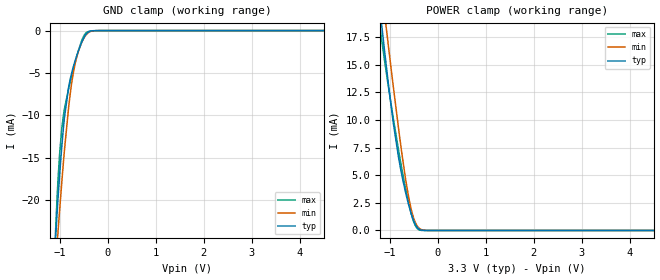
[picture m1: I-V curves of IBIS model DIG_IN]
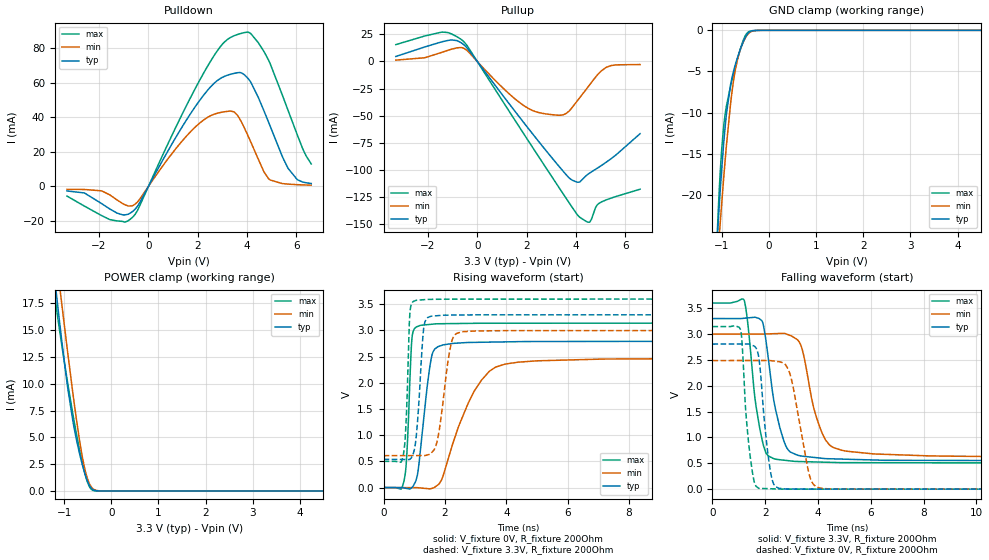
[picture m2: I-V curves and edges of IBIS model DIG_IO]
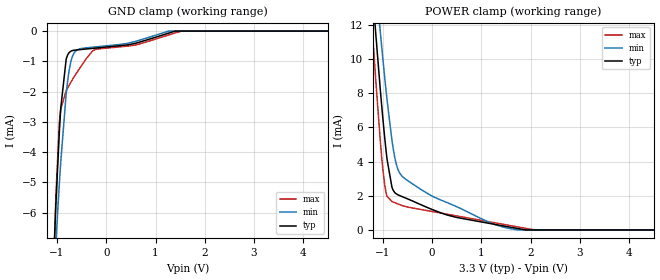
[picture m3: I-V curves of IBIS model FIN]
|Texas Instruments Incorporated
| 13.5 GHz Low Phase Noise Fractional N PLL with Ramp/Chirp Generation
| Part#   Digital Voltage Range   Package-type   #pins
| LMX2492Q   3.0V - 3.6V   PQFP   24
[IBIS Ver]   4.1
[File name]   lmx2492q.ibs
[File Rev]   1.0
[Date]   03/11/2014
[Source]
| Texas Instruments Incorporated.
| 12500 TI Blvd
| Dallas, TX -75243
[Notes]   Revision History:
| Rev 1.0: 03/11/2014
| - Initial version of the model
| - Model generated from simulations in TISPICE
| - C_comp although listed in numerical order of value are
|   obtained from varying PVT conditions. For PVT conditions for
|   each specific value refer the buffer description under
|   respective [Model]. IBIS model user is responsible for using
|   appropriate C_comp to simulate for Signal Integrity.
| - Warnings regarding combined Non-monotonicity of various models have been
|   reviewd and considered minor and can be ignored.
[Disclaimer]
| This model is designed as an aid for customers of Texas Instruments.
| TI and its licensors and suppliers make no warranties, either expressed
| or implied, with respect to this  model, including the warranties of
| merchantability or fitness for a particular purpose. The model is
| provided solely on an "as is" basis. The entire risk as to its quality
| and performance is with the customer.
[Copyright]
 (C) Copyright 2014 Texas Instruments Incorporated.All rights reserved.
|   Device
[Component]   LMX2492Q
[Manufacturer]   TI
[Package]
|   typ   min   max
R_pkg   0.059   0.001   0.103
L_pkg   0.973nH   0.053nH   1.510nH
C_pkg   0.152pF   0.045pF   0.443pF
[Pin]  signal_name   model_name   R_pin   L_pin   C_pin
1   GND   GND   0.01038   0.24453nH   0.44261pF
2   GND   GND   0.04004   0.85295nH   0.16244pF
3   GND   GND   0.03591   0.72509nH   0.15115pF
4   FIN   FIN   0.03459   0.68477nH   0.14617pF
5   FINB   FIN   0.03606   0.72733nH   0.15055pF
6   VCC   POWER   0.0381   0.7937nH   0.13996pF
7   VCC   POWER   0.07708   1.08883nH   0.11244pF
8   VCC   POWER   0.03517   0.70585nH   0.14831pF
9   OSCIN   OSCIN   0.0344   0.682nH   0.14316pF
10   GND/OSCINB   OSCIN   0.03546   0.71302nH   0.14755pF
11   GND   GND   0.03943   0.83863nH   0.16155pF
12   MOD   DIG_IN   0.08857   1.28064nH   0.12455pF
13   CE   DIG_IN   0.09089   1.31884nH   0.12112pF
14   CLK   DIG_IN   0.08649   1.24445nH   0.13324pF
15   DATA   DIG_IN   0.08379   1.20047nH   0.1315pF
16   LE   DIG_IN   0.08521   1.22327nH   0.13399pF
17   MUXOUT   NC   0.09367   1.36085nH   0.1475pF
18   VCC   POWER   0.10259   1.50974nH   0.14764pF
19   VCC   POWER   0.05533   1.28786nH   0.18478pF
20   TRIG1   DIG_IO   0.09611   1.39945nH   0.14699pF
21   TRIG2   DIG_IO   0.08598   1.23277nH   0.13216pF
22   VCP   NC   0.04223   0.89164nH   0.16473pF
23   RESET   NC   0.00048   0.05285nH   0.04508pF
24   CPOUT   NC   0.09024   1.30174nH   0.11914pF
[Diff Pin]  inv_pin  vdiff  tdelay_typ tdelay_min tdelay_max
4   5   200mV   NA   NA   NA
9   10   200mV   NA   NA   NA
| Models and submodels in the file (4): DIG_IN (Input), DIG_IO (I/O), FIN (Input), OSCIN (Input)
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|   Model
[Model]   DIG_IN
Model_type   Input
Vinl = 0.99
Vinh = 2.31
|   typ   min   max
C_comp   0.587pF   0.575pF   0.600pF
[Voltage Range]   3.3   3   3.6
[Temperature Range]   40   125   -40
[Power Clamp Reference]   3.3   3   3.6
[GND Clamp Reference]   0   0   0
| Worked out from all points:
|   GND clamp passes 1 mA (typ) near -0.51 V on its own axis
|   POWER clamp passes 1 mA (typ) near -0.51 V on its own axis
[GND Clamp]
|   Voltage   I(typ)   I(min)   I(max)
-3.3V     -297.7mA   -233.9mA   -460mA
-1.122V   -27.61mA   -30.37mA   -27.79mA
-1.063V   -21.94mA   -25.59mA   -20.2mA
-1.043V   -20.17mA   -24.04mA   -18.04mA
-1.003V   -16.87mA   -21.02mA   -14.41mA
-924mV    -11.35mA   -15.37mA   -9.934mA
-815.1mV  -6.595mA   -8.904mA   -6.77mA
-745.8mV  -4.825mA   -5.878mA   -5.149mA
-607.2mV  -2.293mA   -2.33mA    -2.24mA
-508.2mV  -929.9uA   -987.9uA   -712.3uA
-419.1mV  -217.3uA   -306.5uA   -139.6uA
6.6V      0A         0A         0A
[POWER Clamp]
|   Voltage   I(typ)   I(min)   I(max)
-3.3V     110mA      105.4mA    115.6mA
-1.201V   19.79mA    23.02mA    18.24mA
-1.181V   19mA       22.28mA    17.59mA
-1.112V   16.29mA    19.69mA    15.41mA
-1.043V   13.68mA    17.13mA    13.35mA
-924mV    9.581mA    12.84mA    10.02mA
-785.4mV  5.785mA    8.103mA    6.409mA
-666.6mV  3.332mA    4.494mA    3.656mA
-567.6mV  1.695mA    2.145mA    1.729mA
-468.6mV  542.9uA    714.2uA    425.5uA
-389.4mV  117.3uA    202.9uA    53.06uA
6.6V      0A         0A         0A
|   Model
[Model]   DIG_IO
Model_type   I/O
Polarity   Non-Inverting
Enable   Active-Low
Vinl = 0.99
Vinh = 2.31
Vmeas = 1.65
Vref = 0
Cref = 1pF
Rref = 10000
|   typ   min   max
C_comp   0.587pF   0.575pF   0.600pF
[Voltage Range]   3.3   3   3.6
[Temperature Range]   40   125   -40
[Pullup Reference]   3.3   3   3.6
[Pulldown Reference]   0   -0   0
[Power Clamp Reference]   3.3   3   3.6
[GND Clamp Reference]   0   0   0
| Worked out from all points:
|   slope of the pulldown table from 0 to 0.495 V, typ, clamps not added: 38.1 ohm
|   slope of the pullup table from 0 to 0.495 V, typ, clamps not added: 32.9 ohm
|   GND clamp passes 1 mA (typ) near -0.51 V on its own axis
|   POWER clamp passes 1 mA (typ) near -0.51 V on its own axis
|   falling waveform, V_fixture 3.3V, R_fixture 200Ohm: 20-80 % time 549ps typ, 665ps min, 428ps max; typ from 3.3 V to 0.543 V
|   rising waveform, V_fixture 0V, R_fixture 200Ohm: 20-80 % time 318ps typ, 1.04ns min, 134ps max; typ from 0 V to 2.8 V
|   rising waveform, V_fixture 3.3V, R_fixture 200Ohm: 20-80 % time 183ps typ, 317ps min, 109ps max; typ from 0.54 V to 3.3 V
|   falling waveform, V_fixture 0V, R_fixture 200Ohm: 20-80 % time 311ps typ, 526ps min, 273ps max; typ from 2.81 V to 0 V
[Pulldown]
|   Voltage   I(typ)   I(min)   I(max)
-3.3V     -2.603mA   -1.68mA    -5.588mA
-2.587V   -3.827mA   -1.765mA   -11.42mA
-1.558V   -13.1mA    -4.934mA   -19.2mA
-676.5mV  -14.87mA   -11.28mA   -18.26mA
1.403V    35.27mA    26.86mA    42.78mA
2.373V    55.2mA     39.75mA    68.93mA
3.472V    65.41mA    43.13mA    87.18mA
4.026V    62.67mA    29.64mA    89.31mA
4.927V    35.17mA    3.815mA    71.28mA
5.669V    10.31mA    1.328mA    43.66mA
6.036V    3.907mA    1.017mA    29.8mA
6.6V      1.701mA    750.3uA    13.03mA
[GND Clamp]
|   Voltage   I(typ)   I(min)   I(max)
-3.3V     -297.7mA   -233.9mA   -460mA
-1.122V   -27.61mA   -30.37mA   -27.79mA
-1.063V   -21.94mA   -25.59mA   -20.2mA
-1.043V   -20.17mA   -24.04mA   -18.04mA
-1.003V   -16.87mA   -21.02mA   -14.41mA
-924mV    -11.35mA   -15.37mA   -9.934mA
-815.1mV  -6.595mA   -8.904mA   -6.77mA
-745.8mV  -4.825mA   -5.878mA   -5.149mA
-607.2mV  -2.293mA   -2.33mA    -2.24mA
-508.2mV  -929.9uA   -987.9uA   -712.3uA
-419.1mV  -217.3uA   -306.5uA   -139.6uA
6.6V      0A         0A         0A
[Pullup]
|   Voltage   I(typ)   I(min)   I(max)
-3.3V     4.581mA    1.231mA    15.53mA
-1.399V   18.31mA    8.702mA    27.1mA
-815.1mV  19.22mA    12.56mA    22.74mA
-567.6mV  15.88mA    12.38mA    18.74mA
1.274V    -38.42mA   -29.45mA   -45.26mA
2.234V    -66.53mA   -45.18mA   -78.97mA
3.462V    -100.8mA   -49.34mA   -121.4mA
4.026V    -111.2mA   -37.23mA   -140.5mA
4.551V    -103.1mA   -21.7mA    -148.2mA
4.867V    -98.46mA   -12.5mA    -132.3mA
5.224V    -93.03mA   -5.481mA   -127.8mA
6.6V      -66.66mA   -2.828mA   -117.9mA
[POWER Clamp]
|   Voltage   I(typ)   I(min)   I(max)
-3.3V     110mA      105.4mA    115.6mA
-1.201V   19.79mA    23.02mA    18.24mA
-1.181V   19mA       22.28mA    17.59mA
-1.112V   16.29mA    19.69mA    15.41mA
-1.043V   13.68mA    17.13mA    13.35mA
-924mV    9.581mA    12.84mA    10.02mA
-785.4mV  5.785mA    8.103mA    6.409mA
-666.6mV  3.332mA    4.494mA    3.656mA
-567.6mV  1.695mA    2.145mA    1.729mA
-468.6mV  542.9uA    714.2uA    425.5uA
-389.4mV  117.3uA    202.9uA    53.06uA
6.6V      0A         0A         0A
[Ramp]
R_load = 200
|   typ   min   max
dV/dt_r   1.681/3.17598e-10   1.49252/1.03626e-09   1.88609/1.33572e-10
dV/dt_f   1.65448/5.45285e-10   1.4305/6.64995e-10   1.85889/4.27475e-10
[Falling Waveform]
V_fixture = 3.3V
V_fixture_min = 3V
V_fixture_max = 3.6V
R_fixture = 200Ohm
C_fixture = 0F
|   Time   V(typ)   V(min)   V(max)
0s        3.3V       3V         3.6V
1.201ns   3.306V     3V         3.657V
1.603ns   3.325V     3V         1.788V
1.894ns   3.235V     3V         927.6mV
2.312ns   1.757V     3.007V     592.2mV
2.953ns   717.9mV    2.971V     546.8mV
3.353ns   642mV      2.78V      533.7mV
4.164ns   596.7mV    1.075V     522.8mV
4.897ns   581.5mV    752.5mV    513mV
20ns      542.5mV    615.8mV    501.9mV
[Rising Waveform]
V_fixture = 0V
V_fixture_min = 0V
V_fixture_max = 0V
R_fixture = 200Ohm
C_fixture = 0F
|   Time   V(typ)   V(min)   V(max)
0s        2.795uV    557.9nV    1.379uV
660.4ps   -6.545mV   -489.1uV   115.6mV
762.6ps   -17.44mV   -564.8uV   697.1mV
927.4ps   3.525mV    -687uV     2.868V
1.189ns   651.7mV    -6.823mV   3.096V
1.489ns   2.236V     -23.75mV   3.115V
1.664ns   2.643V     6.019mV    3.125V
2.953ns   2.773V     1.838V     3.137V
3.96ns    2.782V     2.358V     3.138V
20ns      2.802V     2.488V     3.143V
[Rising Waveform]
V_fixture = 3.3V
V_fixture_min = 3V
V_fixture_max = 3.6V
R_fixture = 200Ohm
C_fixture = 0F
|   Time   V(typ)   V(min)   V(max)
0s        540.1mV    609.7mV    500.9mV
637.2ps   536.1mV    610.7mV    609.1mV
733.4ps   535.4mV    610.9mV    1.265V
856.9ps   541.8mV    611.1mV    3.331V
1.044ns   872.5mV    611.4mV    3.573V
1.304ns   3.03V      611.8mV    3.588V
1.541ns   3.271V     653.6mV    3.595V
2.215ns   3.294V     2.78V      3.599V
2.52ns    3.296V     2.971V     3.599V
20ns      3.3V       3V         3.6V
[Falling Waveform]
|Gnd
V_fixture = 0V
V_fixture_min = 0V
V_fixture_max = 0V
R_fixture = 200Ohm
C_fixture = 0F
|   Time   V(typ)   V(min)   V(max)
0s        2.805V     2.488V     3.145V
1.07ns    2.808V     2.488V     3.075V
1.398ns   2.802V     2.488V     772.9mV
1.753ns   2.559V     2.488V     17.18mV
2.18ns    400.3mV    2.488V     8.649mV
2.502ns   19.22mV    2.467V     3.468mV
2.928ns   3.656mV    2.243V     1.038mV
3.671ns   1.325mV    274.4mV    992.7uV
4.047ns   1.295mV    24.22mV    970uV
20ns      13.47uV    557.9nV    6.278uV
|   Model
[Model]   FIN
Model_type   Input
Vinl = 0.99
Vinh = 2.31
|   typ   min   max
C_comp   0.160pF   0.152pF   0.163pF
[Voltage Range]   3.3   3   3.6
[Temperature Range]   40   125   -40
[Power Clamp Reference]   3.3   3   3.6
[GND Clamp Reference]   0   0   0
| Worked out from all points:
|   GND clamp passes 1 mA (typ) near -0.82 V on its own axis
[GND Clamp]
|   Voltage   I(typ)   I(min)   I(max)
-3.3V     -136.1mA   -93.46mA   -260.8mA
-1.063V   -7.299mA   -8.158mA   -7.731mA
-1.043V   -6.485mA   -7.56mA    -6.499mA
-1.023V   -5.706mA   -6.976mA   -5.423mA
-953.7mV  -3.337mA   -5.057mA   -3.029mA
-933.9mV  -2.786mA   -4.551mA   -2.697mA
-815.1mV  -930.7uA   -2.083mA   -1.971mA
-706.2mV  -655.4uA   -931.2uA   -1.654mA
-597.3mV  -622.6uA   -626.7uA   -1.368mA
-260.7mV  -568.5uA   -529.8uA   -638uA
1.531V    0A         0A         0A
6.6V      0A         0A         0A
[POWER Clamp]
|   Voltage   I(typ)   I(min)   I(max)
-3.3V     104.4mA    96.65mA    115.5mA
-1.241V   15.12mA    17.73mA    12.91mA
-1.142V   11.39mA    14.44mA    8.672mA
-1.053V   8.232mA    11.61mA    5.23mA
-963.6mV  5.419mA    8.946mA    2.65mA
-914.1mV  4.114mA    7.58mA     1.966mA
-815.1mV  2.494mA    5.235mA    1.664mA
-755.7mV  2.182mA    4.208mA    1.591mA
-607.2mV  1.949mA    3.137mA    1.428mA
-122.1mV  1.344mA    2.183mA    1.143mA
1.541V    188uA      103.6uA    280.9uA
6.6V      0A         0A         0A
